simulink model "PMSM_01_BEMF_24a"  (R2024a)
settings: Solver=ode45  StartTime=0.0  StopTime=0.1  RelTol=1e-3  EnableMultiTasking=on
undefined symbols (not defined in the file): by, established, Flux, linkage, magnets, V
libraries: spsVoltageMeasurementLib x4, spsSeriesRLCBranchLib x3, spsPermanentMagnetSynchronousMachineLib x1, spspowerguiLib x1

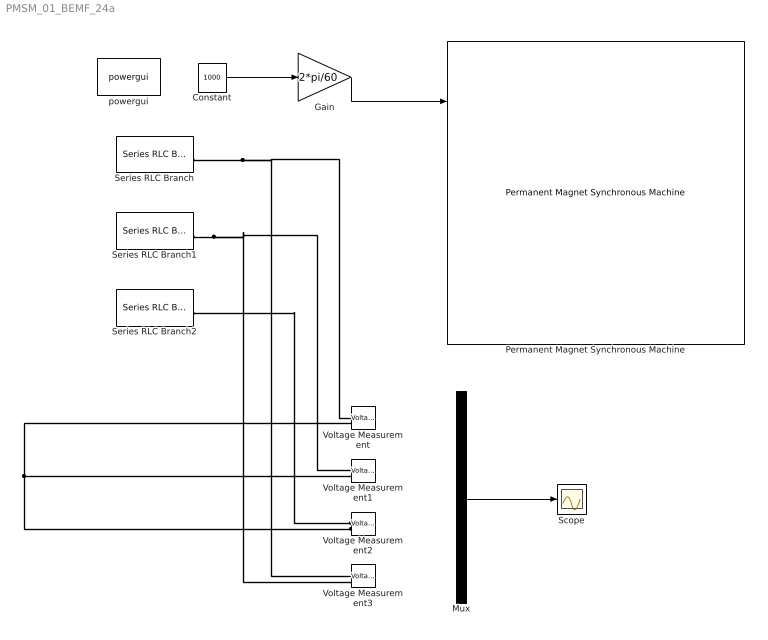
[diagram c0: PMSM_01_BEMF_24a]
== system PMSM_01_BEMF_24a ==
  Constant : Constant  Value=1000
  Gain : Gain  Gain=2*pi/60
  Mux : Mux
  Permanent Magnet Synchronous Machine : spsPermanentMagnetSynchronousMachineLib/Permanent Magnet Synchronous Machine  NbPhases=3  FluxDistribution=Sinusoidal  RotorType=Round  MechanicalLoad=Speed w  PresetModel=No  ShowDetailedParameters=on  MeasurementBus=off  Resistance=0.423  Inductance=8.5e-3  dqInductances=[8.5e-3,8.5e-3]  La=0.00476  MachineConstant=Flux linkage established by magnets (V.s)  Flux=0.422  VoltageCst=153.0847  TorqueCst=1.266  Flat=120  Mechanical=[0.03 0.04 4 0]  PolePairs=2  InitialConditions=[0,0, 0,0]  InitialConditions5ph=[0 0 0 0 0 0]  RefAngle=Aligned with phase A axis (original Park)  IterativeDiscreteModel=Trapezoidal non iterative  TsBlock=-1  TsPowergui=0
  Scope : Scope
  Series RLC Branch : spsSeriesRLCBranchLib/Series RLC Branch  LConnTagsString=__new0  RConnTagsString=__new0  BranchType=R  Resistance=10000  Inductance=1e-3  SetiL0=off  InitialCurrent=0  Capacitance=1e-6  Setx0=off  InitialVoltage=0  Measurements=None
  Series RLC Branch1 : spsSeriesRLCBranchLib/Series RLC Branch  LConnTagsString=__new0  RConnTagsString=__new0  BranchType=R  Resistance=10000  Inductance=1e-3  SetiL0=off  InitialCurrent=0  Capacitance=1e-6  Setx0=off  InitialVoltage=0  Measurements=None
  Series RLC Branch2 : spsSeriesRLCBranchLib/Series RLC Branch  LConnTagsString=__new0  RConnTagsString=__new0  BranchType=R  Resistance=10000  Inductance=1e-3  SetiL0=off  InitialCurrent=0  Capacitance=1e-6  Setx0=off  InitialVoltage=0  Measurements=None
  Voltage Measurement{,1..3} (4 alike) : spsVoltageMeasurementLib/Voltage Measurement  PhasorSimulation=off  OutputType=Complex  PSBequivalent=0
  powergui : spspowerguiLib/powergui  Priority=1  SimulationMode=Continuous  SampleTime=50e-6  frequency=60  Iterations=50  frequencyindice=0  Pbase=100e6  ErrMax=1e-4  UnitsV=kV  UnitsW=MW  buscounter=0  FunctionMessages=off  echomessages=off  EnableUseOfTLC=off  CurrentSourceSwitches=off  DisableSnubberDevices=on  DisableRonSwitches=on  DisableVfSwitches=on  DisplayEquations=off  AutomaticDiscreteSolvers=off  SolverType=Tustin  Interpol=off  ExternalGateDelay=off  methode=off  Ts=0  x0status=blocks  SPID=on  SwTol=0  HookPort=off  NonlinearTolerance=1e-4  nMaxIteration=100  ContinueOnMaxIteration=off  RestoreLinks=warning  ResistiveCurrentMeasurement=off  Frange=[0:2:500]  Ylog=off  Xlog=on  ShowGrid=off  save=off  variable=ZData  structure=0  ZoomFFT=off  StartTime=0.0  cycles=1  DisplayStyle=1  fundamental=60  FreqAxis=off  MaxFrequency=1000  frequencyindicesteady=1  RmsSteady=1  display=off
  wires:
  Gain/1 -> Permanent Magnet Synchronous Machine/1
  Constant/1 -> Gain/1
  Mux/1 -> Scope/1
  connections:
  Series RLC Branch/RConn1 -- Voltage Measurement/LConn1 -- Voltage Measurement3/LConn1
  Series RLC Branch1/RConn1 -- Voltage Measurement1/LConn1 -- Voltage Measurement3/LConn2
  Voltage Measurement2/LConn1 -- Series RLC Branch2/RConn1
  Voltage Measurement2/LConn2 -- Voltage Measurement/LConn2 -- Voltage Measurement1/LConn2
